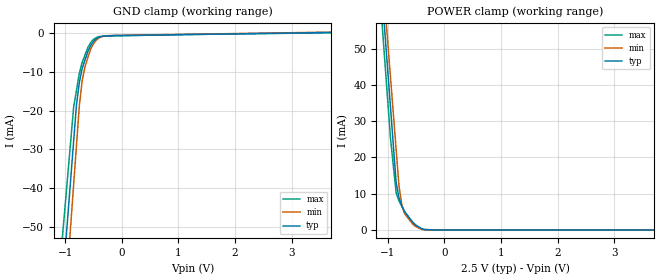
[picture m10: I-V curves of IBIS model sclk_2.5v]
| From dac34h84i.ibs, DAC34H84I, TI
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[Model] sclk_2.5v
Model_type Input
Vinl = 750.000mV
Vinh = 1.75000V
C_comp 641.000fF 640.000fF 642.000fF
| variable typ   min   max
[Voltage Range] 2.50000V 2.25000V 2.75000V
[POWER Clamp Reference] 2.50000V 2.25000V 2.75000V
[GND Clamp Reference] 0.00000V 0.00000V 0.00000V
[Temperature Range] 25   125   -40
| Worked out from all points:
|   GND clamp passes 1 mA (typ) near -0.41 V on its own axis
|   POWER clamp passes 1 mA (typ) near -0.47 V on its own axis
[GND Clamp]
-2.5V     -338.8mA   -374.2mA   -299mA
-850mV    -27.88mA   -39.1mA    -19.05mA
-800mV    -18.46mA   -28.95mA   -14.69mA
-750mV    -12.71mA   -18.79mA   -10.34mA
-700mV    -9.123mA   -12.3mA    -7.518mA
-650mV    -6.903mA   -8.636mA   -5.594mA
-600mV    -4.682mA   -6.34mA    -3.671mA
-550mV    -3.127mA   -4.044mA   -2.38mA
-450mV    -1.33mA    -1.739mA   -1.06mA
-350mV    -723.9uA   -789.2uA   -774.1uA
-150mV    -564.1uA   -502.4uA   -625.2uA
5V        541.8uA    638.1uA    420.2uA
[POWER Clamp]
-2.5V     356.1mA    352.5mA    355.6mA
-1.1V     65.06mA    72.22mA    57.28mA
-1.05V    54.67mA    62.21mA    46.62mA
-950mV    33.88mA    42.19mA    25.31mA
-850mV    13.09mA    22.16mA    10.2mA
-800mV    8.915mA    12.15mA    8.016mA
-750mV    6.545mA    7.011mA    6.529mA
-700mV    5.051mA    4.458mA    5.043mA
-550mV    2.022mA    1.494mA    1.963mA
-400mV    375.9uA    171.3uA    241.9uA
-175mV    0A         0A         25.38uA
5V        0A         0A         0A
